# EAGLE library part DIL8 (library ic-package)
Dual In Line / Socket
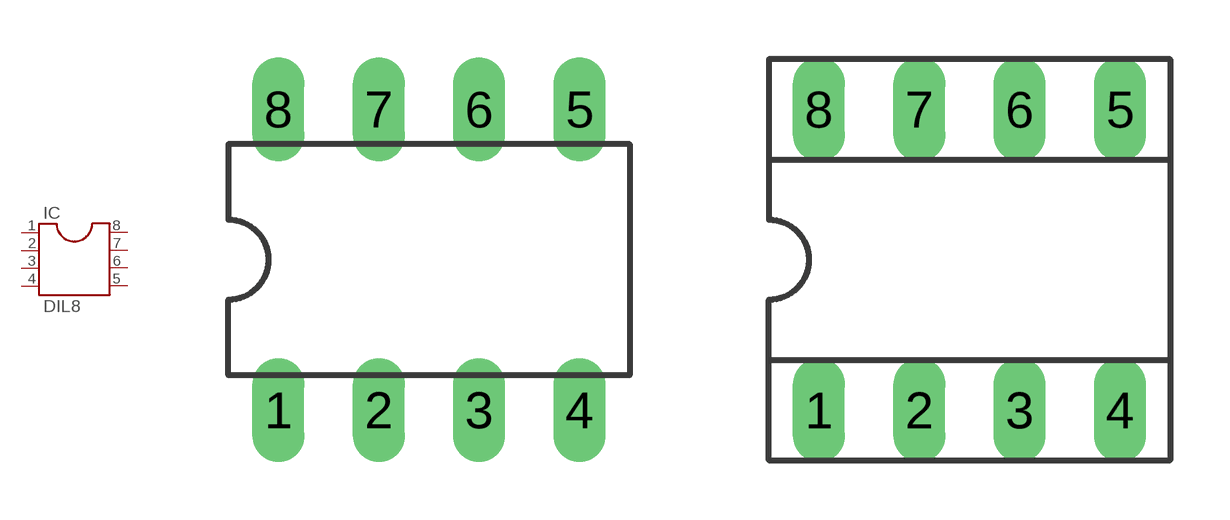
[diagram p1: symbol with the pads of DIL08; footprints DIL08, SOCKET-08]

Designator prefix IC

## DIL8  [DIL08]
1  1  pas
2  2  pas
3  3  pas
4  4  pas
5  5  pas
6  6  pas
7  7  pas
8  8  pas

## DIL8S  [SOCKET-08]
Pads as for DIL08

## Footprint DIL08 (pad centres in mm)
Dual In Line Package
drill 0.813 long: 1 -3.81,-3.81; 2 -1.27,-3.81; 3 1.27,-3.81; 4 3.81,-3.81; 5 3.81,3.81; 6 1.27,3.81; 7 -1.27,3.81; 8 -3.81,3.81

## Footprint SOCKET-08 (pad centres in mm)
Dual In Line Socket
drill 0.813 long: 1 -3.81,-3.81; 2 -1.27,-3.81; 3 1.27,-3.81; 4 3.81,-3.81; 5 3.81,3.81; 6 1.27,3.81; 7 -1.27,3.81; 8 -3.81,3.81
